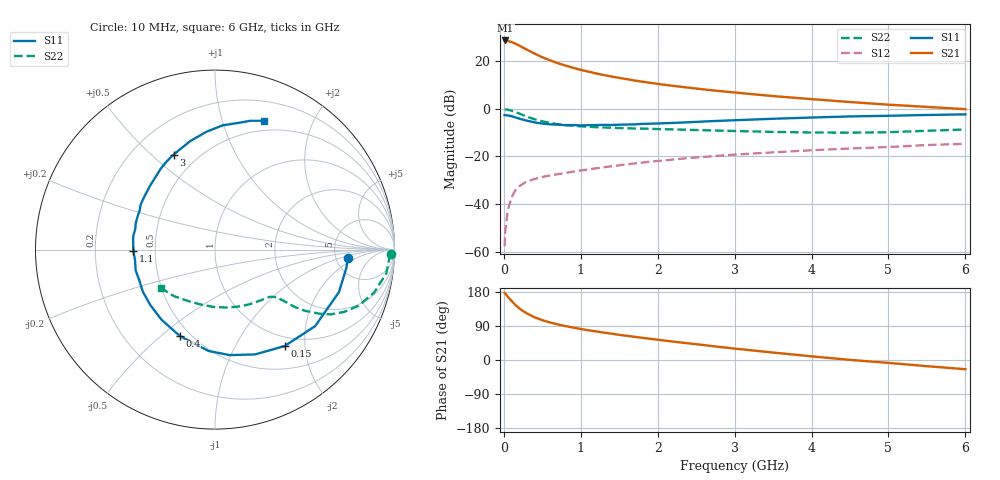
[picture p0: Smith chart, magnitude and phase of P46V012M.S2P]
! SIEMENS Small Signal Semiconductors
! BFP182
! Si NPN RF Bipolar Junction Transistor in SOT143
! VCE = 6 V  IC = 12 mA
! Common Emitter S-Parameters:  March  1996
# GHz  S  MA  R  50
!  f  S11  S21  S12  S22
! GHz  MAG  ANG  MAG  ANG  MAG  ANG  MAG  ANG
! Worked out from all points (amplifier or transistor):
!   36 points, 10 MHz to 6 GHz, reference 50 ohm
!   highest |S21| = 28.8 dB at 20 MHz (marker M1)
!   |S21| within 3 dB of that: start of sweep to 248 MHz
!   unconditionally stable (mu >= 1): 1.146 GHz to 5.472 GHz
!   at 250 MHz: K = 0.35, MSG = 28.6 dB, |S12| = -31.5 dB
!   at 1.4 GHz: K = 1.08, MAG = 17.2 dB, |S12| = -24.1 dB
!   at 6 GHz: K = 0.95, MSG = 7.3 dB, |S12| = -14.7 dB
!   S11 on the Smith chart (normalised r, x): 10 MHz: 6.42, -1.36; 150 MHz: 0.84, -1.62; 400 MHz: 0.44, -0.58; 1.1 GHz: 0.38, -0.01; 3 GHz: 0.37, +0.59; 6 GHz: 0.39, +1.37
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0.01  0.7408 -3.7  27.39 177.1  0.0013 80.9  0.9789 -1.5
0.02  0.7393 -7.8  27.46 175.0  0.0028 90.0  0.9722 -3.1
0.05  0.7302 -18.9  26.95 167.3  0.0073 82.3  0.9634 -7.9
0.1  0.7022 -37.4  25.33 155.8  0.0138 71.4  0.9176 -15.2
0.15  0.6627 -54.2  23.48 145.3  0.0194 65.9  0.8596 -21.3
0.2  0.6252 -69.1  21.43 136.4  0.0236 60.4  0.7982 -25.8
0.25  0.5934 -82.1  19.36 129.0  0.0267 56.2  0.7393 -29.2
0.3  0.5661 -93.6  17.61 123.0  0.0298 53.0  0.6844 -31.5
0.4  0.5201 -112.1  14.5 112.7  0.0336 49.5  0.604 -34.3
0.5  0.4912 -127.5  12.15 105.1  0.0371 46.6  0.5474 -35.7
0.6  0.4745 -139.5  10.54 99.0  0.0399 46.2  0.5064 -36.3
0.7  0.4656 -149.7  9.134 94.0  0.0424 46.1  0.4779 -36.7
0.9  0.4568 -165.4  7.319 85.7  0.048 46.2  0.442 -37.4
1.1  0.4543 -178.8  6.067 78.3  0.0535 46.9  0.4208 -38.8
1.5  0.4653 161.8  4.48 66.4  0.0651 47.0  0.396 -42.5
1.8  0.4834 149.1  3.739 58.5  0.0742 46.2  0.3848 -46.4
2.2  0.5071 135.6  3.048 48.6  0.0862 44.3  0.3706 -52.6
3  0.5774 113.6  2.212 30.2  0.1093 38.8  0.3428 -68.0
3.5  0.62 102.9  1.859 19.6  0.122 35.0  0.3282 -79.5
4.5  0.6945 86.3  1.393 0.3  0.1468 27.1  0.3162 -105.5
5.5  0.7445 74.6  1.101 -16.3  0.1737 19.8  0.3465 -131.8
6  0.7673 69.3  0.987 -24.3  0.1845 15.1  0.3689 -144.4
